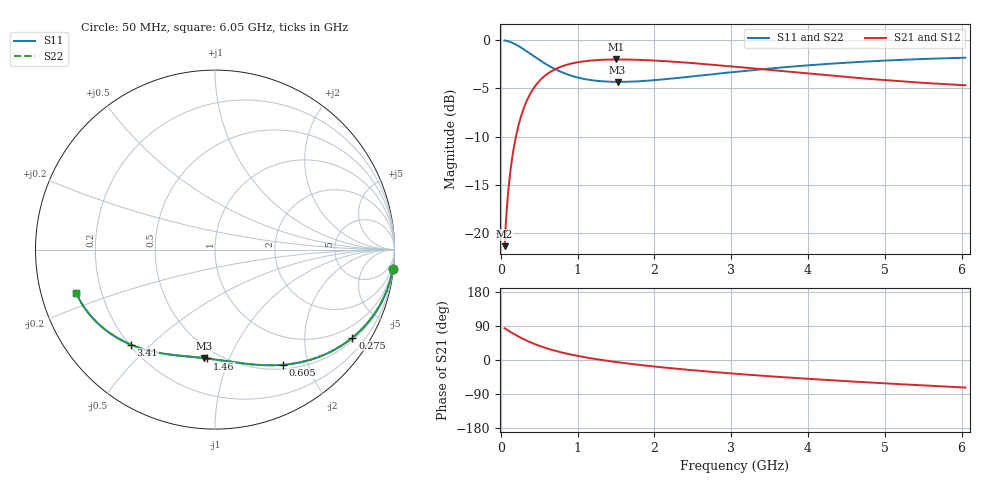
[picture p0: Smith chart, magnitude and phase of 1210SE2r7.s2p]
! AVX Thin Film Operation		Date: August 2001
! Description: Accu-P® Series, Thin Film, SMD, RF Capacitor
! Part Number: 12101J2R7ABT
! 50 MHz  -  6.05 GHz
! Serial Measurements
# mhz S db R 50
!	S11		S21		S12		S22
!	dB	Phase	dB	Phase	dB	Phase	dB	Phase
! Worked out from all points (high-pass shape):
!   401 points, 50 MHz to 6.05 GHz, reference 50 ohm
!   highest |S21| = -2.00 dB at 1.505 GHz (marker M1); lowest = -21.4 dB at 50 MHz (marker M2)
!   |S21| within 3 dB of the highest: 427.1 MHz to end of sweep
!   lowest |S11| = -4.3 dB at 1.52 GHz (marker M3), VSWR 4.09, Z = 21.2 - j40.5 ohm
!   |S11| at or under -10 dB: nowhere
!   |S22| runs from -4.3 to 0.0 dB; largest |S21 - S12| = 0
!   S11 on the Smith chart (normalised r, x): 50 MHz: 1, -18; 275 MHz: 0.59, -3.32; 605 MHz: 0.56, -1.60; 1.46 GHz: 0.43, -0.83; 3.41 GHz: 0.20, -0.43; 6.05 GHz: 0.11, -0.15
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50  -0.03 -6.4  -21.36 83.6  -21.36 83.6  -0.03 -6.4
65  -0.05 -8.3  -19.11 81.7  -19.11 81.7  -0.05 -8.3
110  -0.15 -13.9  -14.67 76.1  -14.67 76.1  -0.15 -13.9
155  -0.29 -19.3  -11.88 70.7  -11.88 70.7  -0.29 -19.3
215  -0.54 -26.2  -9.36 63.8  -9.36 63.8  -0.54 -26.2
275  -0.83 -32.7  -7.62 57.3  -7.62 57.3  -0.83 -32.7
350  -1.23 -40.0  -6.09 50.0  -6.09 50.0  -1.23 -40.0
425  -1.64 -46.6  -5.03 43.4  -5.03 43.4  -1.64 -46.6
605  -2.56 -59.6  -3.51 30.4  -3.51 30.4  -2.56 -59.6
815  -3.39 -71.1  -2.66 18.9  -2.66 18.9  -3.39 -71.1
1055  -3.97 -81.3  -2.23 8.7  -2.23 8.7  -3.97 -81.3
1250  -4.22 -88.0  -2.07 2.0  -2.07 2.0  -4.22 -88.0
1460  -4.32 -94.2  -2.01 -4.2  -2.01 -4.2  -4.32 -94.2
1505  -4.33 -95.4  -2.00 -5.4  -2.00 -5.4  -4.33 -95.4
1520  -4.33 -95.8  -2.00 -5.8  -2.00 -5.8  -4.33 -95.8
2060  -4.11 -108.5  -2.14 -18.5  -2.14 -18.5  -4.11 -108.5
2525  -3.73 -117.4  -2.40 -27.4  -2.40 -27.4  -3.73 -117.4
3050  -3.29 -126.2  -2.76 -36.2  -2.76 -36.2  -3.29 -126.2
3410  -3.01 -131.6  -3.02 -41.6  -3.02 -41.6  -3.01 -131.6
4055  -2.58 -140.3  -3.50 -50.3  -3.50 -50.3  -2.58 -140.3
5060  -2.10 -152.2  -4.18 -62.3  -4.18 -62.3  -2.10 -152.2
6050  -1.82 -162.7  -4.67 -72.8  -4.67 -72.8  -1.82 -162.7
